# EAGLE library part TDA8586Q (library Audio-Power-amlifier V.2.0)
Power amplifier with load detection and auto BTL/SE selection
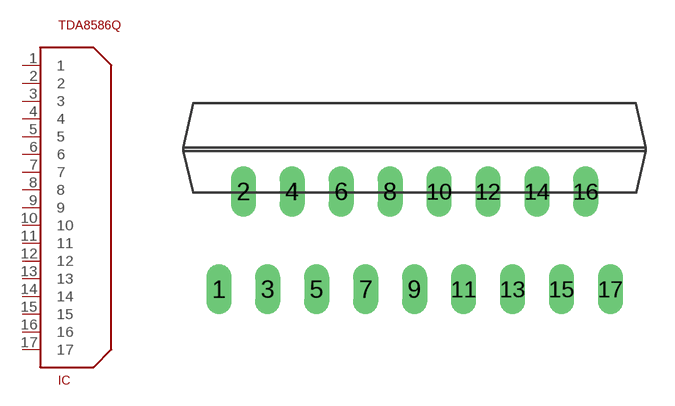
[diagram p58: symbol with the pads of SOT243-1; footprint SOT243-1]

Designator prefix IC

## TDA8586Q  [SOT243-1]
1  1  out
2  2  pwr
3  3
4  4  out
5  5  in
6  6  in
7  7  in
8  8  in
9  9  pwr
10  10  pwr
11  11
12  12
13  13
14  14  out
15  15
16  16  pwr
17  17  out

## Footprint SOT243-1 (pad centres in mm)
DBS17P: plastic DIL-bent-SIL power package; 17 leads (lead length 7.7 mm)
drill 0.8 long: 1 -10.16,-5.08; 2 -8.89,0; 3 -7.62,-5.08; 4 -6.35,0; 5 -5.08,-5.08; 6 -3.81,0; 7 -2.54,-5.08; 8 -1.27,0; 9 0,-5.08; 10 1.27,0; 11 2.54,-5.08; 12 3.81,0; 13 5.08,-5.08; 14 6.35,0; 15 7.62,-5.08; 16 8.89,0; 17 10.17,-5.08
